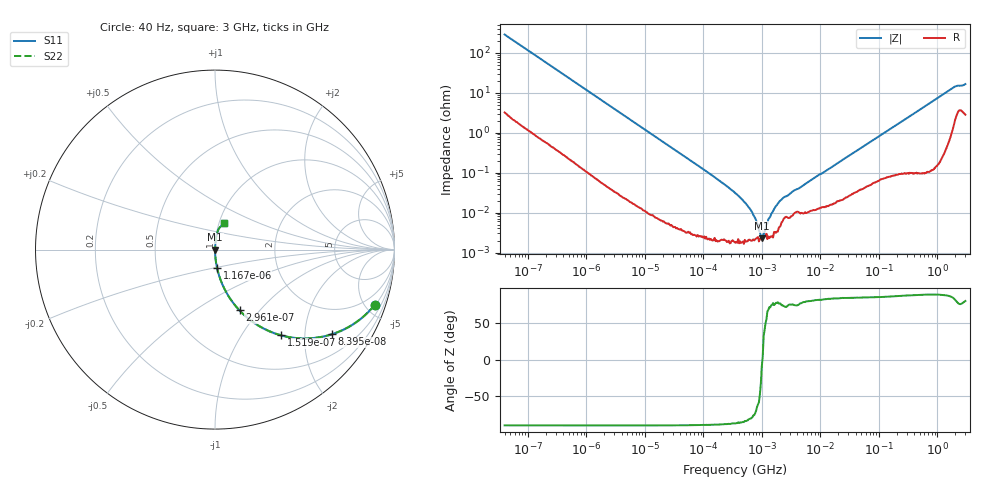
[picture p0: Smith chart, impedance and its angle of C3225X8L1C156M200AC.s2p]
! S-Parameter Data Generated by TDK Corporation
! Copyright(C) 2024 TDK Corporation.
! All Rights Reserved.
! TDK P/N: C3225X8L1C156M200AC (Multilayer Ceramic Chip Capacitor)
! Property: C=15uF
! Size(LxWxT): 3.2x2.5x2mm
! Model Type: s2p (Touchstone File Format Version 1.0)
! Frequency: DC=Yes Start=4E-05MHz Stop=3000MHz 622points Log-sweep
! Model Generated on May 28, 2024
! Terms and conditions regarding TDK Simulation Models:
! 1)This simulation model is being provided solely for informational
!  purposes. Please refer to the specifications of the products in
!  terms of detailed characteristics of such products.
! 2)In no event shall TDK Corporation of any of its subsidiaries be
!  liable for any loss or damage arising, directly or indirectly,
!  from any information contained in this simulation model, including,
!  but not limited to loss or damages arising from any inaccuracies,
!  omissions or errors in connection with such information.
! 3)Any and all copyrights on this simulation model are owned by
!  TDK Corporation.  Duplication or redistribution of this simulation
!  model without prior written permission from TDK Corporation
!  is prohibited.
! 4)This simulation model is subject to any modification or change
!  without any prior notice.
! 5)Neither TDK Corporation nor any of its subsidiaries shall make any
!  warranty, express or implied, including but not limited to the
!  correctness, implied warranties of merchantability and fitness for
!  a particular purpose with respect to this simulation models.
! 6)The use of this simulation model shall be deemed to have consented
!  to the terms and conditions hereof.
! Port Assignments:
!  1 ---| |--- 2
! Applicable Conditions:
!  Temperature = 25 degC
!  DC Bias Voltage = 0 V
!  Small Signal Operation
# Hz S MA R 50
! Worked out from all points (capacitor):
!   621 points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, 40 Hz to 3 GHz, reference 50 ohm
!   read as one part in series: C = 13.9 uF near 44.7 Hz
!   lowest |Z| = 2.28 mohm at 992.9 kHz (marker M1)
!   series resonance near 1.019 MHz, so ESL is about 1.8 nH
!   S11 on the Smith chart (normalised r, x): 40 Hz: 1.06, -5.73; 83.95 Hz: 1.03, -2.75; 151.9 Hz: 1.01, -1.52; 296.1 Hz: 1.01, -0.79; 1.167 kHz: 1.00, -0.20; 3 GHz: 1.06, +0.32
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40  0.9409 -19.2  0.3282 70.2  0.3282 70.2  0.9409 -19.2
57.949  0.8886 -26.7  0.4495 62.7  0.4495 62.7  0.8886 -26.7
83.951  0.8045 -35.9  0.586 53.6  0.586 53.6  0.8045 -35.9
151.915  0.6034 -52.3  0.7916 37.1  0.7916 37.1  0.6034 -52.3
296.053  0.3651 -68.0  0.9274 21.4  0.9274 21.4  0.3651 -68.0
461.902  0.2453 -75.3  0.9671 14.2  0.9671 14.2  0.2453 -75.3
835.84  0.1396 -81.5  0.989 8.0  0.989 8.0  0.1396 -81.5
1166.832  0.1009 -83.7  0.994 5.8  0.994 5.8  0.1009 -83.7
3418.691  0.03494 -87.5  0.9991 2.0  0.9991 2.0  0.03494 -87.5
17465.72  0.00691 -89.0  0.9999 0.4  0.9999 0.4  0.00691 -89.0
134151.2  0.0008935 -88.5  1 0.1  1 0.1  0.0008935 -88.5
351682.9  0.0003045 -86.7  1 0.0  1 0.0  0.0003045 -86.7
685363.9  9.989e-05 -78.4  1 0.0  1 0.0  9.989e-05 -78.4
765977.9  7.269e-05 -72.9  1 0.0  1 0.0  7.269e-05 -72.9
992897.8  2.275e-05 -9.5  1 0.0  1 0.0  2.275e-05 -9.5
1438427  9.16e-05 74.2  1 -0.0  1 -0.0  9.16e-05 74.2
2244233  0.0002245 74.5  0.9999 -0.0  0.9999 -0.0  0.0002245 74.5
7348767  0.0006911 80.6  0.9999 -0.0  0.9999 -0.0  0.0006911 80.6
1.49005e8  0.01174 85.5  0.9991 -0.7  0.9991 -0.7  0.01174 85.5
6.296259e8  0.04723 86.1  0.9979 -2.7  0.9979 -2.7  0.04723 86.1
1.855641e9  0.1309 76.8  0.9785 -7.5  0.9785 -7.5  0.1309 76.8
3e9  0.158 71.2  0.9608 -9.0  0.9608 -9.0  0.158 71.2
